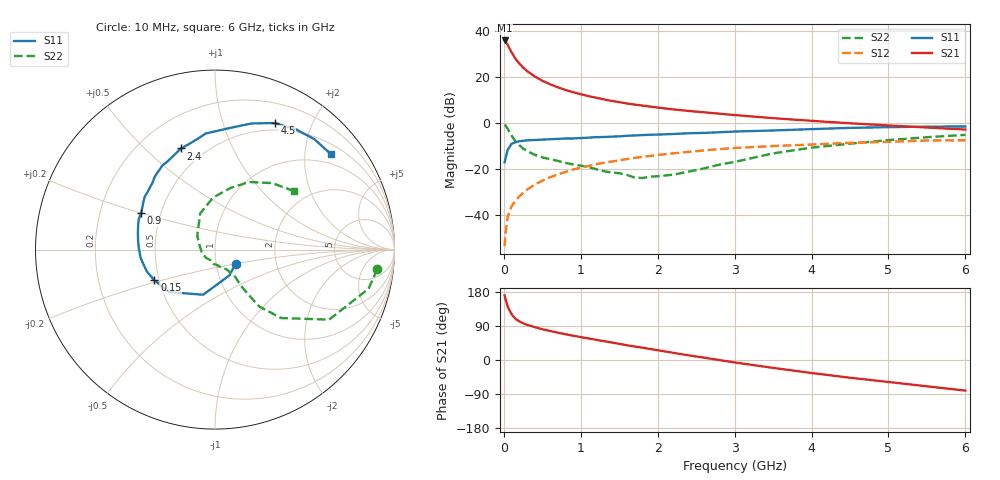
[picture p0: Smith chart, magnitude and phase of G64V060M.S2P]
! SIEMENS Small Signal Semiconductors
! BFG193
! Si NPN RF Bipolar Junction Transistor in SOT223
! VCE = 4 V  IC = 60 mA
! Common Emitter S-Parameters:  August  1996
# GHz  S  MA  R  50
!  f  S11  S21  S12  S22
! GHz  MAG  ANG  MAG  ANG  MAG  ANG  MAG  ANG
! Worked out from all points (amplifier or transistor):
!   36 points, 10 MHz to 6 GHz, reference 50 ohm
!   highest |S21| = 35.8 dB at 10 MHz (marker M1)
!   |S21| within 3 dB of that: start of sweep to 66.58 MHz
!   unconditionally stable (mu >= 1): 391.8 MHz to 2.346 GHz
!   at 250 MHz: K = 0.94, MSG = 27.2 dB, |S12| = -30.4 dB
!   at 1.4 GHz: K = 1.05, MAG = 11.9 dB, |S12| = -16.8 dB
!   at 6 GHz: K = 0.90, MSG = 2.3 dB, |S12| = -7.6 dB
!   S11 on the Smith chart (normalised r, x): 10 MHz: 1.24, -0.20; 150 MHz: 0.47, -0.19; 900 MHz: 0.39, +0.20; 2.4 GHz: 0.37, +0.65; 4.5 GHz: 0.42, +1.49; 6 GHz: 0.73, +2.60
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0.01  0.1395 -34.6  61.68 170.5  0.0021 90.7  0.9108 -6.9
0.02  0.1647 -60.8  59.12 162.4  0.0038 79.7  0.8827 -14.3
0.05  0.2599 -104.7  49.27 140.9  0.0092 70.4  0.7463 -31.5
0.1  0.35 -137.5  34.23 120.9  0.0153 69.1  0.5304 -46.0
0.15  0.3784 -153.3  24.91 108.8  0.0203 67.8  0.4018 -52.1
0.2  0.3991 -162.3  19.59 102.1  0.0252 69.8  0.3292 -53.1
0.25  0.4077 -168.9  15.92 96.9  0.0302 70.1  0.2766 -53.9
0.3  0.4169 -173.6  13.46 92.9  0.0353 70.5  0.2471 -54.3
0.4  0.425 178.7  10.24 86.9  0.0455 70.2  0.2031 -53.7
0.5  0.433 172.2  8.226 81.1  0.0555 69.6  0.178 -53.2
0.6  0.4407 167.0  6.907 76.6  0.0657 68.5  0.163 -54.3
0.7  0.4493 162.4  5.942 72.2  0.076 67.1  0.1497 -56.7
0.9  0.4589 153.8  4.638 64.1  0.0968 63.3  0.1248 -60.2
1.1  0.4782 146.7  3.813 56.9  0.1156 59.6  0.1095 -70.0
1.3  0.4938 139.7  3.237 49.7  0.1361 55.4  0.0893 -79.2
1.6  0.5246 130.1  2.638 38.9  0.1639 48.6  0.0739 -102.9
2.2  0.5731 113.6  1.963 19.1  0.218 35.0  0.0748 -168.7
2.4  0.5945 108.6  1.818 12.3  0.2346 30.7  0.0872 166.9
3.5  0.6836 82.8  1.266 -20.8  0.3142 3.5  0.2175 112.3
4.5  0.7792 64.8  0.98 -46.8  0.3688 -16.5  0.3529 76.1
5.5  0.8276 48.0  0.793 -69.4  0.4141 -40.0  0.4886 49.3
6  0.8362 39.6  0.716 -80.8  0.4191 -53.4  0.5486 36.4
